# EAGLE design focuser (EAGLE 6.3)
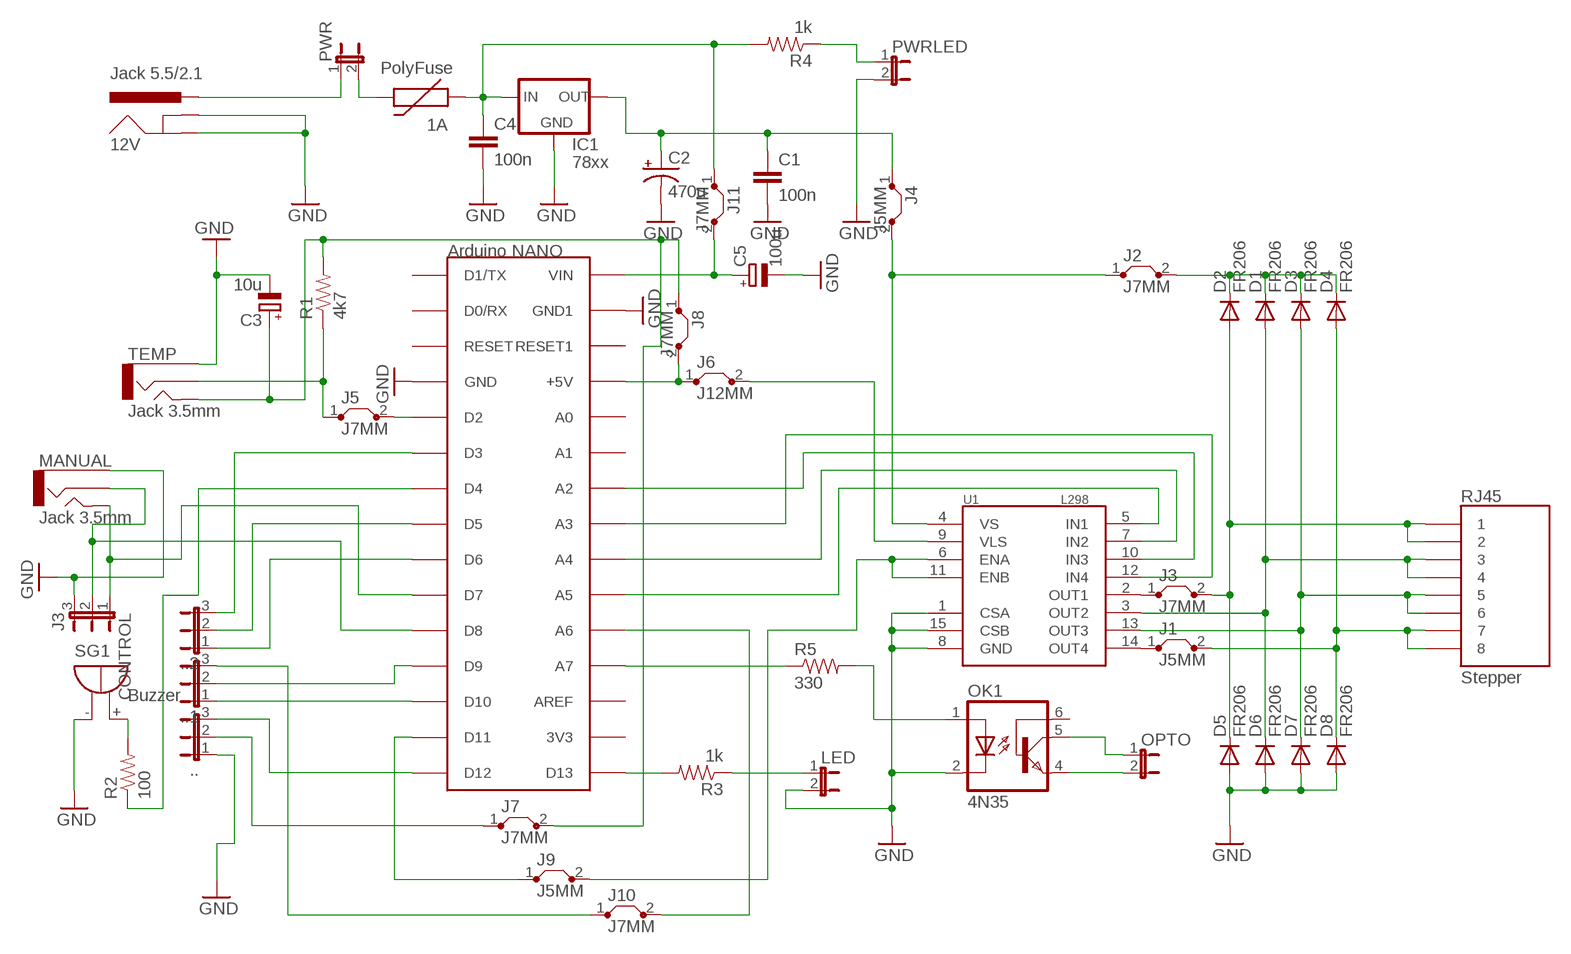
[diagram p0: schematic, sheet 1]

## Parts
1A  PolyFuse  PTCPTH  [PTC]
12V  Jack 5.5/2.1  POWER_JACKCOMBO  [POWER_JACK_COMBO]
..  JUMPER-3PTH  [1X03]
..1  JUMPER-3PTH  [1X03]
..2  JUMPER-3PTH  [1X03]
C1  100n  CAP_  [AXIAL-5MM]
C2  470u  CAP_POLPTH1  [CPOL-RADIAL-100UF-25V]
C3  10u  CPOL-EUE2-4  [E2-4]
C4  100n  CAP_  [AXIAL-5MM]
C5  100u  CPOL-EUE2-4  [E2-4]
CONTROL  J3  JUMPER-3PTH  [1X03]
D1  FR206  DIODEPTH  [DIODE-1N4001]
D2  FR206  DIODEPTH  [DIODE-1N4001]
D3  FR206  DIODEPTH  [DIODE-1N4001]
D4  FR206  DIODEPTH  [DIODE-1N4001]
D5  FR206  DIODEPTH  [DIODE-1N4001]
D6  FR206  DIODEPTH  [DIODE-1N4001]
D7  FR206  DIODEPTH  [DIODE-1N4001]
D8  FR206  DIODEPTH  [DIODE-1N4001]
IC1  78xx  V_REG_78XXSINK  [TO220-IGO]
J1  J5MM  [05]
J2  J7MM  [07]
J3  J7MM  [07]
J4  J5MM  [05]
J5  J7MM  [07]
J6  J12MM  [12]
J7  J7MM  [07]
J8  J7MM  [07]
J9  J5MM  [05]
J10  J7MM  [07]
J11  J7MM  [07]
LED  JUMPER-2PTH  [1X02]
MANUAL  Jack 3.5mm  AUDIO-JACKPTH  [AUDIO-JACK]
NANO  MMduino  ARDUINONANO  [PDIP-32]
OK1  4N35  [DIL06]
OPTO  JUMPER-2PTH  [1X02]
PWR  JUMPER-2PTH  [1X02]
PWRLED  JUMPER-2PTH  [1X02]
R1  4k7  RESISTORPTH1  [AXIAL-0.3]
R2  100  RESISTORPTH1  [AXIAL-0.3]
R3  1k  RESISTORPTH1  [AXIAL-0.3]
R4  1k  RESISTORPTH1  [AXIAL-0.3]
R5  330  RESISTORPTH1  [AXIAL-0.3]
RJ45  Stepper  RJ45-8PTH  [RJ45-8]
SG1  Buzzer  F/QMBIII  [F/QMBIII]
TEMP  Jack 3.5mm  AUDIO-JACKPTH  [AUDIO-JACK]
U1  L298  [MULTIWATT15]

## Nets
+5: C3.+ J7.2 J8.1 R1.P$2 TEMP.5
GND [power]: 12V.GND(GNDBREAK) 12V.GND@1(GND) ...1 C1.P$2 C2.2(-) C3.- C4.P$2 C5.- CONTROL.3 D5.A D6.A D7.A D8.A IC1.GND LED.2 MANUAL.1 NANO.GND NANO.GND1 OK1.2(C) PWRLED.2 SG1.-(+) TEMP.1 U1.1(CSA) U1.8(GND) U1.15(CSB)
N$2: J6.2 U1.9(VLS)
N$3: J9.2 U1.6(ENA) U1.11(ENB)
N$4: NANO.A5 U1.5(IN1)
N$5: NANO.A4 U1.7(IN2)
N$6: ...2 J7.1
N$7 [power]: 1A.P$2 PWR.2
N$8 [power]: CONTROL.2 MANUAL.2 NANO.D8
N$9 [power]: 1A.P$1 C4.P$1 IC1.IN J11.1 R4.P$2
N$10 [power]: D4.A D8.C J1.2 RJ45.7 RJ45.8
N$11: J1.1 U1.14(OUT4)
N$12: NANO.A7 R5.P$1
N$13: NANO.A2 U1.10(IN3)
N$14 [power]: D1.A D6.C RJ45.3 RJ45.4 U1.3(OUT2)
N$15: NANO.A3 U1.12(IN4)
N$16 [power]: D2.A D5.C J3.2 RJ45.1 RJ45.2
N$17: J5.1 R1.P$1 TEMP.2
N$18: ..1.2 NANO.D9
N$19: J5.2 NANO.D2
N$20 [power]: PWRLED.1 R4.P$1
N$21 [power]: D3.A D7.C RJ45.5 RJ45.6 U1.13(OUT3)
N$22 [power]: D1.C D2.C D3.C D4.C J2.2
N$23: J3.1 U1.2(OUT1)
N$24: R2.P$2 SG1.+(-)
N$25: ...3 NANO.D12
N$27 [power]: J2.1 J4.2 U1.4(VS)
N$28: NANO.D13 R3.P$2
N$29: LED.1 R3.P$1
N$30: 12V.POWER(PWR) PWR.1
N$31: ..1.1 NANO.D10
N$32: ..2.3 NANO.D3
N$33: NANO.D4 R2.P$1
N$34: ..2.2 NANO.D5
N$35: ..2.1 NANO.D6
N$37: OK1.1(A) R5.P$2
N$38: OK1.4(EMI) OPTO.2
N$39: OK1.5(COL) OPTO.1
N$40: CONTROL.1 MANUAL.5 NANO.D7
N$41: J10.2 NANO.A6
N$42: J9.1 NANO.D11
N$43: ..1.3 J10.1
N$44 [power]: C5.+ J11.2 NANO.VIN
N$45: J6.1 J8.2 NANO.+5V
VCC2 [power]: C1.P$1 C2.1(+) IC1.OUT J4.1
Unconnected: NANO.3V3 NANO.A0 NANO.A1 NANO.AREF NANO.D0/RX NANO.D1/TX NANO.RESET NANO.RESET1 OK1.6(BAS)

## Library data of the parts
1A = SparkFun:PTC: Resettable Fuse PTC
12V = SparkFun:POWER_JACK: Power Jack This is the standard 5.5mm barrel jack for power. The PTH is the most common, proven, reliable, footprint. All others are experimental. The Slot footprint only works if the mill layer is transmitted to the PCB fab house so be warned. Spark Fun Electronics SKU : PRT-00119. Mating wall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
.. ..1 ..2 CONTROL = SparkFun:JUMPER-3
C1 C4 = SparkFun:CAP: Capacitor
C2 = SparkFun:CAP_POL: Capacitor Polarized
C3 C5 = resistor:CPOL-EU: POLARIZED CAPACITOR, European symbol
D1-D8 = SparkFun:DIODE: Diode
IC1 = SparkFun:V_REG_78XX: Voltage Regulator Standard 7805 5V regulator. IGO (Input Ground Output). Spark Fun Electronics SKU : COM-00107
J1-J11 = jumper:J: Bridge
LED OPTO PWR PWRLED = SparkFun:JUMPER-2: Jumper
MANUAL TEMP = SparkFun:AUDIO-JACK: 3.5mm Audio Jack Simple 3.5mm common PCB mount audio jack. SKU: PRT-08032
NANO = jet-lib:ARDUINONANO; NAM: Arduino NANO
OK1 = optocoupler:4N35: MOTOROLA OPTO COUPLER; MF: FAIRCHILD SEMICONDUCTOR; MPN: 4N35; OC_FARNELL: 1328375; OC_NEWARK: 72K9946
R1-R5 = SparkFun:RESISTOR: Resistor
RJ45 = SparkFun:RJ45-8: RJ45 Jack Simple RJ45, 8-pin connection - connector for common Cat5, Cat5e, and Cat6 Ethernet cables. Footprint not yet proven in production. Connector sku is PRT-00643; Breakout PCB sku is BOB-00716.
SG1 = buzzer2:F/QMBIII: BUZZER; OC_FARNELL: unknown; OC_NEWARK: unknown
U1 = SparkFun:L298: L298 Dual Full Bridge Driver

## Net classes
0 default: width 0.254 mm, drill 0.635 mm, clearance 0.203 mm
1 power: width 0.254 mm, drill 0.635 mm, clearance 0.203 mm

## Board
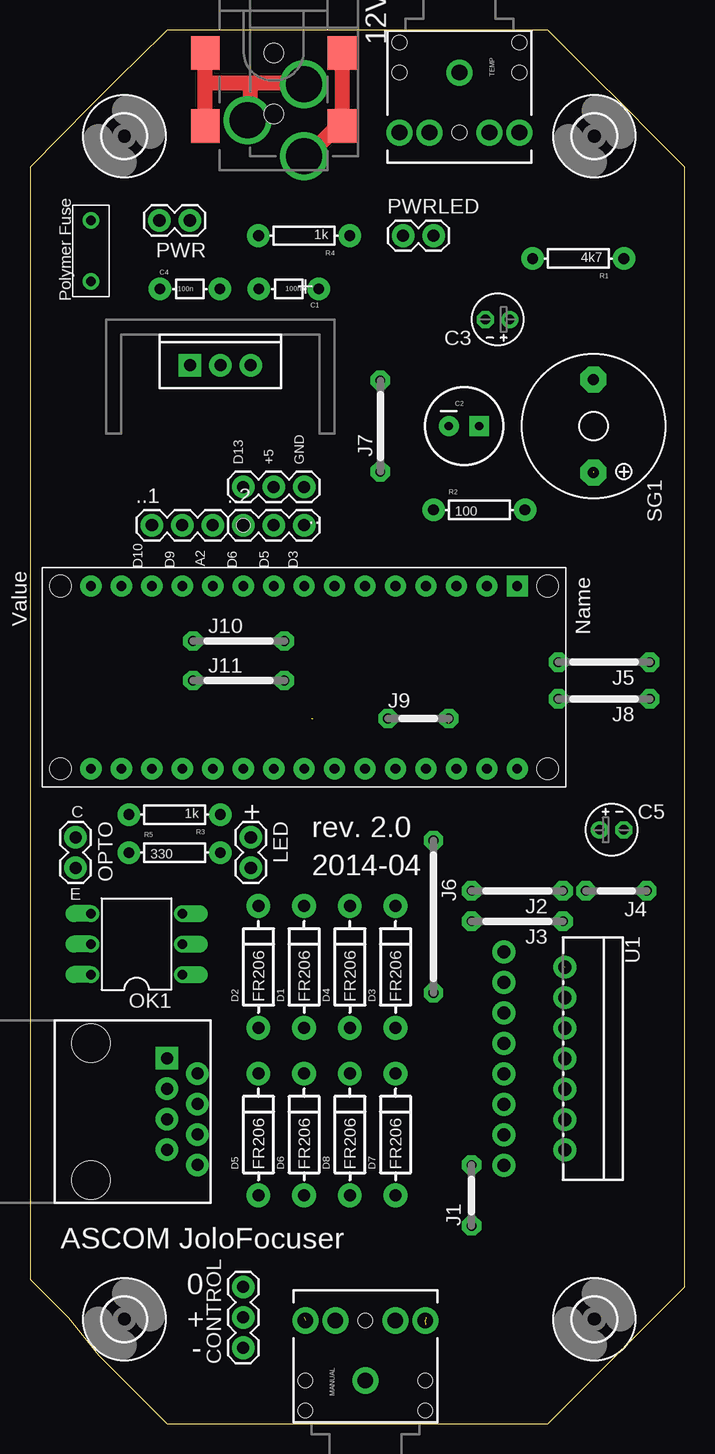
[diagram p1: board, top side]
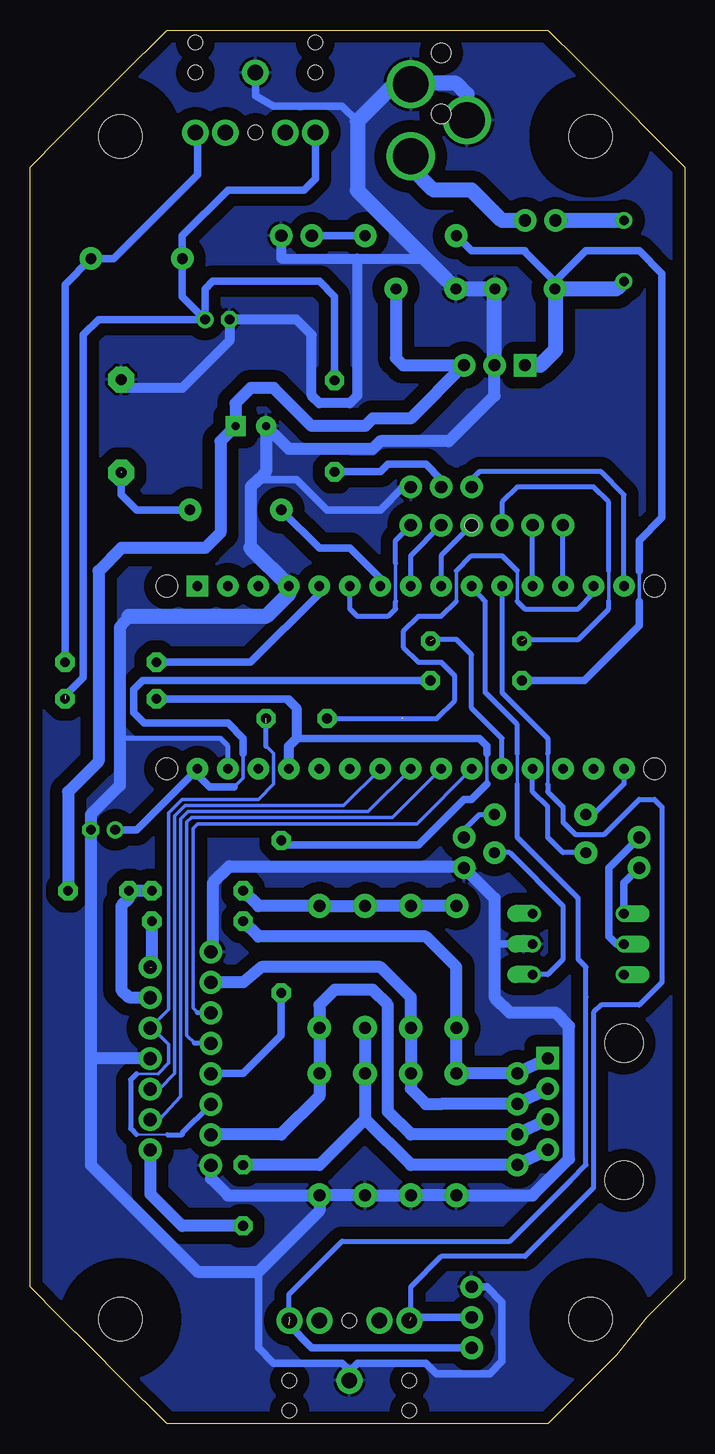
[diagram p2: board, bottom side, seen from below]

Size 54.61 x 116.21 mm. Coordinates in mm from the lower left corner, seen from the top.
Outline: 5.71,5.71 11.43,0 43.18,0 46.99,3.81 49.51,6.35 52.07,8.89 54.61,11.43 54.61,104.78 52.07,107.32 49.51,109.91 46.99,112.4 43.18,116.21 11.43,116.21 8.89,113.67 7.62,112.45 5.08,109.91 2.54,107.32 0,104.78 0,12.07 3.17,8.89 5.71,5.71
Copper layers (1*16): Top 0.035mm / dielectric 1.5mm / Bottom 0.035mm
Design rules "SparkFun": minimum track width 8mil, minimum drill 20mil, track to track 8mil, track to pad 8mil, pad to pad 8mil, via to via 8mil, smd to smd 8mil, copper to edge 10mil, drill to drill 8mil, minimum pad ring 12mil, minimum via ring 10mil, stop-mask expansion 4mil, vias tented up to drill 25mil, thermal gap 10mil
Holes 1.1 mm at 17.78,74.93

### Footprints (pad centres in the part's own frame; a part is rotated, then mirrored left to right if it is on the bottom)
PTC = drill 0.8: P$1 -2.54,0; P$2 2.54,0
POWER_JACK_COMBO = drill 2.997: GND 5.62,-2.16; GND@1 2.62,2.54; POWER 8.62,2.54 | smd 2.8 x 2.4: GND@3 0,-5.7; GND@4 6.1,-5.7; POWER@1 0,5.7; POWER@2 6.1,5.7 | hole 1.6: 0,0; 5.08,0
1X03 = drill 1.016 pad 1.88: 1 0,0; 2 2.54,0; 3 5.08,0
AXIAL-5MM = drill 0.9 pad 1.88: P$1 -2.5,0; P$2 2.5,0
CPOL-RADIAL-100UF-25V = drill 0.7 pad 1.651 square: 1 1.27,0 | drill 0.7 pad 1.651: 2 -1.27,0
E2-4 = drill 0.813 pad 1.27: + -1.016,0 | drill 0.813 pad 1.27 octagon: - 1.016,0
DIODE-1N4001 = drill 1 pad 1.981: A -5.08,0; C 5.08,0
TO220-IGO = drill 1 pad 1.88: GND 0,0; OUT 2.54,0 | drill 1 pad 1.88 square: IN -2.54,0
05 = drill 0.813 pad 1.6 octagon: 1 -2.54,0; 2 2.54,0
07 = drill 0.813 pad 1.6 octagon: 1 -3.81,0; 2 3.81,0
12 = drill 0.813 pad 1.6 octagon: 1 -6.35,0; 2 6.35,0
1X02 = drill 1.016 pad 1.88: 1 0,0; 2 2.54,0
AUDIO-JACK = drill 1.3 pad 2.184: 1 0,0; 2 5,5; 3 5,2.5; 4 5,-2.5; 5 5,-5 | hole 1.2: 0,5; -2.5,5; -2.5,-5; 0,-5; 5,0
PDIP-32 = drill 0.8 pad 1.778: 3V3 15.24,-35.56; +5V 15.24,-10.16; A0 15.24,-12.7; A1 15.24,-15.24; A2 15.24,-17.78; A3 15.24,-20.32; A4 15.24,-22.86; A5 15.24,-25.4; A6 15.24,-27.94; A7 15.24,-30.48; AREF 15.24,-33.02; D0/RX 0,-5.08; D2 0,-12.7; D3 0,-15.24; D4 0,-17.78; D5 0,-20.32; D6 0,-22.86; D7 0,-25.4; D8 0,-27.94; D9 0,-30.48; D10 0,-33.02; D11 0,-35.56; D12 0,-38.1; D13 15.24,-38.1; GND 0,-10.16; GND1 15.24,-5.08; RESET 0,-7.62; RESET1 15.24,-7.62; VIN 15.24,-2.54 | drill 0.8 pad 1.778 square: D1/TX 0,-2.54 | hole 1.778: 0,0; 0,-40.64; 15.24,-40.64; 15.24,0
DIL06 = drill 0.813 offset: 1 -2.54,-3.81; 2 0,-3.81; 3 2.54,-3.81; 4 2.54,3.81; 5 0,3.81; 6 -2.54,3.81
AXIAL-0.3 = drill 0.9 pad 1.88: P$1 -3.81,0; P$2 3.81,0
RJ45-8 = drill 1 pad 1.88 square: 1 -4.445,6.35 | drill 1 pad 1.88: 2 -3.175,8.89; 3 -1.905,6.35; 4 -0.635,8.89; 5 0.635,6.35; 6 1.905,8.89; 7 3.175,6.35; 8 4.445,8.89 | hole 3.2: -5.715,0; 5.715,0
F/QMBIII = drill 0.914 pad 2.159 octagon: + 3.886,0; - -3.886,0
MULTIWATT15 = drill 1.1 pad 1.9: 1 -8.95,-2.39; 2 -7.68,2.69; 3 -6.41,-2.39; 4 -5.14,2.69; 5 -3.87,-2.39; 6 -2.6,2.69; 7 -1.33,-2.39; 8 -0.06,2.69; 9 1.21,-2.39; 10 2.48,2.69; 11 3.75,-2.39; 12 5.02,2.69; 13 6.29,-2.39; 14 7.56,2.69; 15 8.83,-2.39
3,6 = hole 3.6: 0,0

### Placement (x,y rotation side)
1A  5.08,97.79 90 top
12V  20.32,114.3 270 top
..  22.86,78.11 180 top
..1  10.16,74.93 0 top
..2  17.78,74.93 0 top
C1  21.59,94.62 180 top
C2  36.2,83.19 0 top
C3  38.99,92.08 180 top
C4  13.33,94.62 0 top
C5  48.51,49.53 0 top
CONTROL  17.78,6.35 90 top
D1  22.86,38.1 90 top
D2  19.05,38.1 90 top
D3  30.48,38.1 90 top
D4  26.67,38.1 90 top
D5  19.05,24.13 90 top
D6  22.86,24.13 90 top
D7  30.48,24.13 90 top
D8  26.67,24.13 90 top
IC1  15.88,88.27 0 top
J1  36.83,19.05 90 top
J2  40.64,44.45 180 top
J3  40.64,41.91 180 top
J4  48.9,44.45 180 top
J5  47.88,63.5 180 top
J6  33.66,42.29 270 top
J7  29.21,83.19 90 top
J8  47.88,60.45 180 top
J9  32.38,58.8 0 top
J10  17.4,65.28 0 top
J11  17.4,61.98 0 top
LED  18.41,48.89 270 top
MANUAL  27.97,3.63 90 top
NANO  43.18,69.85 270 top
OK1  8.89,40.01 90 top
OPTO  3.81,48.89 270 top
PWR  13.33,100.33 180 top
PWRLED  31.11,99.06 0 top
R1  45.72,97.16 180 top
R2  37.47,76.2 0 top
R3  12.06,50.8 180 top
R4  22.86,99.06 180 top
R5  12.06,47.62 0 top
RJ45  5.08,26.04 270 top
SG1  46.99,83.19 270 top
TEMP  35.81,112.65 270 top
U1  41.91,30.4 270 top
U$2  [3,6]  7.87,8.74 0 top
U$3  [3,6]  47.07,8.74 0 top
U$4  [3,6]  47.07,107.34 0 top
U$5  [3,6]  7.87,107.34 0 top

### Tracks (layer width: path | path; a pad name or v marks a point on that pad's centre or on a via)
+5  (1 unrouted)
  Bottom 0.61: J7.2 29.21,93.98 30.48,95.25 39.37,95.25 40.01,94.62 C3.+ | 51.69,60.71 50.17,62.23 50.17,90.81 48.9,92.08 C3.+ | C3.+ 41.91,93.98 R1.P$2 41.91,99.06 38.1,102.87 31.75,102.87 30.81,103.81 TEMP.5
GND
  Bottom 0.406: NANO.GND1 38.1,56.52 38.74,57.15 47.12,57.15 | 21.63,97.16 19.7,95.23
  Bottom 0.61: OK1.2 15.88,40.01 | 35.56,78.74 32.38,78.74 29.84,76.2 25.4,76.2 23.5,78.11 ...1 | TEMP.1 35.81,110.74 34.29,109.86 28.57,109.86 27.3,108.59 | 35.56,12.7 35.56,6.35 34.29,5.08 28.57,5.08 27.94,4.45 27.3,5.08 21.59,5.08 20.7,4.19 16.26,4.19 15.24,5.21 15.24,10.16 16.51,11.43 CONTROL.3
  Bottom 0.813: PWRLED.2 33.66,97.16 27.3,97.16 | SG1.- 46.91,86.36 41.91,86.36 37.97,90.3 C3.- 32.38,92.08 31.11,90.81 31.11,85.73 30.48,85.09 27.94,85.09 27.3,85.73 27.3,97.16 | 27.3,97.16 21.63,97.16
  Bottom 1.016: U1.15 39.52,20.47 38.1,19.05 D7.A | 49.53,30.48 C5.- 49.53,50.8 47.12,53.21 47.12,57.15 47.12,66.42 46.36,67.31 | 49.53,30.48 49.53,21.59 40.64,12.7 35.56,12.7 30.48,17.78 D7.A | 18.29,46.48 37.97,46.48 39.37,45.09 39.37,39.37 | U1.8 49.51,30.46 49.53,30.48 | D7.A D8.A D6.A D5.A 12.7,19.05 9.65,22.1 9.65,33.15 10.79,34.29 14.61,34.29 15.88,35.56 15.88,40.01 15.88,43.81 LED.2 | NANO.GND 33.02,69.22 | 36.2,73.03 36.2,78.11 35.56,78.74 34.93,79.38 C2.2 33.02,81.28 26.04,81.28 25.4,81.92 19.68,81.92 15.88,85.73 IC1.GND
  Bottom 1.27: 33.02,69.22 34.93,67.31 46.36,67.31 | 36.2,73.03 NANO.GND | 12V.GND 18.16,110.87 19.05,111.76 22.78,111.76 12V.GND@1 24.21,111.68 27.3,108.59 27.3,102.83 19.7,95.23 C1.P$2 C4.P$2 15.88,94.58 IC1.GND
  pour Bottom (isolate 1.016): 0,0 0,116.21 54.61,116.21 54.61,0
N$2
  Bottom 0.305: 39.5,29.21 U1.9
  Bottom 0.61: J6.2 33.66,32.38 36.83,29.21 39.5,29.21
N$3  (1 unrouted)
  Bottom 0.203: 43.94,29.18 45.72,29.18 | 45.73,24.11 43.18,24.13 43.16,24.11
  Bottom 0.254: 41.91,24.11 41.91,24.26
  Bottom 0.305: 43.94,29.18 43.05,30.1 43.05,31.62 44.43,33 U1.6 43.05,34.55 43.05,50.93 41.91,52.07 35.56,52.07 34.29,53.34 34.29,55.88 34.93,56.52
  Bottom 0.406: 45.72,29.18 46.23,28.7 46.23,24.64 45.73,24.11 | 43.16,24.11 41.91,24.11 | 41.91,24.26 U1.11 | 34.93,56.52 34.93,58.42
N$4
  Bottom 0.305: 40.64,34.29 41.02,34.67 41.02,49.66 40.64,50.04 22.35,50.04 NANO.A5 | 39.54,34.29 U1.5
  Bottom 0.406: 40.64,34.29 39.54,34.29
N$5
  Bottom 0.305: 40.89,31.75 41.53,32.38 41.53,50.16 41.15,50.55 24.38,50.55 NANO.A4 | 39.54,31.75 U1.7
  Bottom 0.406: 40.89,31.75 39.54,31.75
N$6
  Bottom 0.61: ...2 20.32,78.74 21.59,80.01 24.77,80.01 25.4,79.38 J7.1
N$7
  Bottom 1.27: 1A.P$2 PWR.2
N$8  (1 unrouted)
  Bottom 0.305: 11.43,55.88 11.43,53.34
  Bottom 0.406: 22.86,8.89 22.86,11.43 20.32,13.97 13.33,13.97 7.62,19.68 7.62,34.29 6.98,34.92 3.81,34.92 1.91,36.83 1.91,51.44 2.54,52.07 3.81,52.07 6.73,49.15 9.14,49.15 10.16,50.16 10.16,51.44 11.43,52.7 11.43,53.34 | NANO.D8 15.24,60.96 11.43,57.15 11.43,55.88
  Bottom 0.61: CONTROL.2 22.86,8.89
N$9
  Bottom 0.305: 3.81,68.58 3.81,71.12
  Bottom 0.61: 3.81,71.12 3.81,73.66 1.91,75.57 1.91,95.89 3.81,97.79 8.26,97.79 10.83,95.21 | 10.83,95.21 C4.P$1 10.79,94.58 | 10.83,95.21 13.33,97.71 13.33,97.79 17.78,97.79 R4.P$2 | 3.81,68.58 3.81,66.55 8.38,61.98 J11.1
  Bottom 1.27: 1A.P$1 5.71,94.62 C4.P$1 | 10.79,94.58 10.79,89.54 12.06,88.27 IC1.IN
N$10
  Bottom 1.016: RJ45.7 RJ45.8 22.86,21.59 26.67,25.4 | 26.67,25.4 30.48,21.59 J1.2 | D4.A D8.C 26.67,25.4
N$11
  Bottom 1.016: J1.1 41.91,16.51 44.58,19.18 U1.14
N$12
  Bottom 0.406: R5.P$1 10.16,47.62 11.43,48.89 11.43,51.44 12.7,52.7 NANO.A7
N$13
  Bottom 0.305: U1.10 44.58,27.94 43.82,27.94 42.55,29.21 42.55,50.67 41.66,51.56 28.45,51.56 NANO.A2
N$14
  Bottom 0.406: 39.5,36.83 U1.3
  Bottom 1.016: RJ45.3 RJ45.4 20.32,26.67 21.59,26.67 22.86,27.94 D6.C D1.A 22.86,35.56 25.4,38.1 35.31,38.1 36.83,36.83 39.5,36.83
N$15
  Bottom 0.305: U1.12 44.58,25.4 43.82,25.4 42.04,27.3 42.04,50.42 41.4,51.05 26.42,51.05 NANO.A3
N$16
  Bottom 1.016: RJ45.1 RJ45.2 D5.C D2.A 19.05,38.1 21.59,40.64 35.56,40.64 J3.2
N$17
  Bottom 0.406: 51.44,63.75 J5.1
  Bottom 0.61: J5.1 51.69,95 R1.P$1 47.62,97.16 40.64,104.14 40.64,107.48 TEMP.2
N$18
  Bottom 0.406: NANO.D9 ..1.2
N$19
  Bottom 0.61: NANO.D2 30.48,69.22 36.2,63.5 J5.2
N$20
  Bottom 0.61: R4.P$1 PWRLED.1
N$21
  Bottom 0.406: 39.5,24.13 U1.13
  Bottom 1.016: RJ45.5 RJ45.6 22.86,24.13 24.77,26.04 24.77,34.92 26.04,36.2 29.21,36.2 30.48,34.92 D3.A D7.C 30.48,27.3 33.66,24.13 39.5,24.13
N$22
  Bottom 1.016: D2.C D1.C D4.C D3.C 35.56,43.18 J2.2
N$23  (1 unrouted)
  Bottom 1.016: J3.1 44.45,38.1
N$24  (1 unrouted)
  Bottom 0.61: R2.P$2 45.72,76.2 46.99,77.47 46.99,79.38
N$25
  Bottom 0.406: NANO.D12 5.08,77.47 6.98,79.38 17.14,79.38 17.78,78.74 ...3
N$27
  Bottom 0.406: J4.2 46.36,43.81 | 44.62,35.56 U1.4
  Bottom 1.016: J2.1 J4.2 | 46.36,43.81 46.99,43.18 46.99,36.2 46.36,35.56 44.62,35.56
N$28
  Bottom 0.406: NANO.D13 5.08,53.34 7.62,50.8 R3.P$2
N$29
  Bottom 0.406: LED.1 18.41,49.53 17.14,50.8 R3.P$1
N$30
  Bottom 1.27: PWR.1 15.24,100.33 17.78,102.87 20.95,102.87 22.86,104.78 12V.POWER
N$31
  Bottom 0.406: NANO.D10 ..1.1
N$32
  Bottom 0.305: 24.13,68.58 24.13,71.76
  Bottom 0.406: 24.13,68.58 24.13,67.95 24.77,67.31 27.3,67.31 27.94,67.95 NANO.D3 | 24.13,71.76 24.13,73.66 ..2.3
  Bottom 0.61: NANO.D3 27.94,69.22
N$33
  Bottom 0.61: NANO.D4 25.4,70.48 27.94,73.03 30.48,73.03 R2.P$1
N$34
  Bottom 0.406: NANO.D5 22.86,72.39 ..2.2
N$35
  Bottom 0.406: ..2.1 20.32,72.39 NANO.D6
N$37
  Bottom 0.406: OK1.1 11.43,37.46 10.16,38.73 10.16,43.18 14.61,47.62 R5.P$2
N$38
  Bottom 0.61: OK1.4 5.08,45.09 OPTO.2
N$39
  Bottom 0.61: OPTO.1 6.35,46.35 6.35,40.64 5.71,40.01 OK1.5
N$40  (2 unrouted)
  Bottom 0.305: 13.97,53.34 13.97,55.88
  Bottom 0.406: 33.02,8.89 33.02,10.8 28.57,15.24 14.61,15.24 9.53,20.32 8.26,21.59 8.26,35.56 8.26,38.1 8.89,38.73 8.89,43.81 13.97,48.89 13.97,53.34 | 13.97,55.88 13.97,58.29 16.64,60.96 16.64,68.58 NANO.D7
  Bottom 0.61: CONTROL.1 31.11,6.35 33.02,8.25
N$41  (1 unrouted)
  Bottom 0.406: NANO.A6 15.24,57.15 17.78,59.69 17.78,64.14 19.05,65.41 20.95,65.41
N$42  (1 unrouted)
  Bottom 0.305: 19.05,68.58 19.05,71.12 | 13.97,71.12 13.97,68.58
  Bottom 0.406: 23.5,58.8 20.7,58.8 19.18,60.32 19.18,62.36 20.32,63.5 22.22,63.5 23.5,64.77 23.5,66.04 22.22,67.31 20.32,67.31 19.05,68.58 | J9.1 23.62,58.8 | 19.05,71.12 17.78,72.39 15.24,72.39 13.97,71.12 | 13.97,68.58 13.33,67.95 8.89,67.95 7.62,69.22 NANO.D11
N$43  (1 unrouted)
  Bottom 0.305: 6.35,68.58 6.35,71.12
  Bottom 0.406: 13.33,65.41 8.89,65.41 6.35,67.95 6.35,68.58 | 6.35,71.12 6.35,76.84 7.62,78.11 13.97,78.11 15.24,76.84 ..1.3
N$44
  Bottom 0.254: NANO.VIN 40.64,54.1
  Bottom 0.305: 37.59,53.09 36.83,53.85 36.83,55.88
  Bottom 0.61: C5.+ 45.72,49.53 NANO.VIN | 40.64,54.1 39.62,53.09 37.59,53.09 | J11.2 45.21,61.98 45.97,61.21 45.97,59.31 45.09,58.42 38.1,58.42 36.83,57.15 36.83,55.88
N$45
  Bottom 0.305: 33.53,48.26 J6.1 | 16.51,53.34 16.51,55.88
  Bottom 0.406: 33.15,60.45 33.02,60.32
  Bottom 0.61: 32.38,57.15 19.68,57.15 17.14,57.15 16.51,56.52 16.51,55.88 | 33.53,48.26 22.22,48.26 19.05,51.44 18.41,52.07 17.78,52.07 16.51,53.34 | 33.15,60.45 J8.2
  Bottom 0.813: NANO.+5V 33.02,56.52 32.38,57.15 32.38,59.69 33.02,60.32
VCC2
  Bottom 1.016: J4.1 51.44,52.7 48.9,55.24 48.9,71.12 46.99,73.03 40.01,73.03 38.74,74.3 38.74,81.92 C2.1 37.47,85.09 36.2,86.36 34.29,86.36 31.11,83.19 26.67,83.19 26.04,83.82 22.86,83.82 IC1.OUT 23.5,88.27 24.09,88.86 C1.P$1

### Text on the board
tNames: Polymer Fuse | + | D13 | +5 | GND | D10 | D9 | A2 | D6 | D5 | D3 | C | + | rev. 2.0 | 2014-04 | E | ASCOM JoloFocuser | 0 | + | -
tValues: ASCOM JoloFocuser

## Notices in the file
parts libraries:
SparkFun: Licensing: CC v3.0 Share-Alike You are welcome to use this library for commercial purposes.
